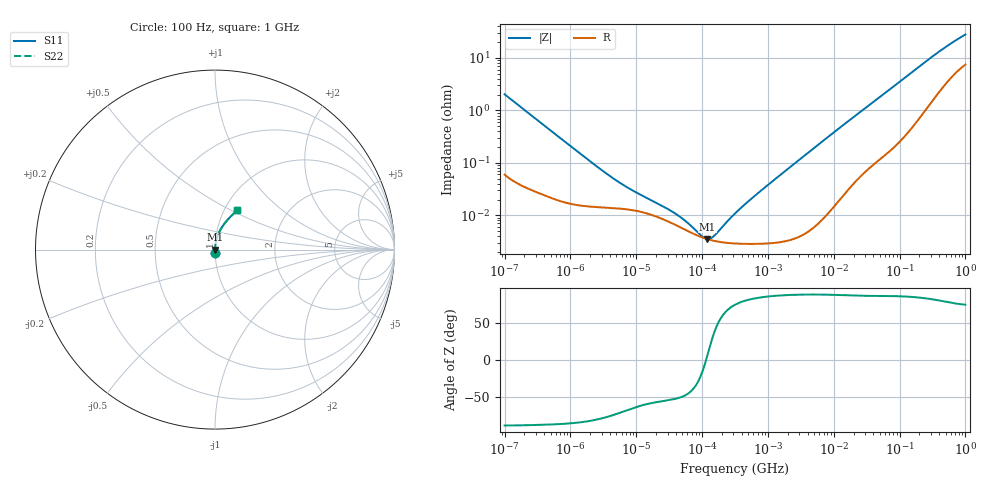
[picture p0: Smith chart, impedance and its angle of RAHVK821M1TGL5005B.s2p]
! RAHVK821M1TGL5005B  S-PARAMETER MODEL  (AEC-Q200 qualified)
! Model Generated by ELNA Corporation (http://www.ty-top.com)
! Version 1.0
! ELNA Control No. 201211
! Copyright (c) 2020 ELNA CO.,LTD. All Rights Reserved.
! Products Name : CONDUCTIVE POLYMER HYBRID ALUMINUM ELECTROLYTIC CAPACITORS
! Characteristics :
!  Capacitance  :  820uF  ,  Rated voltage  :  25V
!  Operating Temp. Range  :  -55 to +125 degC  ,  Endurance  :  6000hr at 125 degC
!  Dimension D  :  12.5mm  ,  Dimension L  :  13.5mm
! Frequency Range : 100Hz - 1GHz
! External Node Assignments :
!  1  o---| |---o  2
# MHz S RI R 50
!Freq[MHz].  S11 Real  S11 Imag  S21 Real  S21 Imag  S12 Real  S12 Imag  S22 Real  S22 Imag
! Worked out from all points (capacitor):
!   401 points, 100 Hz to 1 GHz, reference 50 ohm
!   read as one part in series: C = 782 uF near 108 Hz
!   lowest |Z| = 3.53 mohm at 120.2 kHz (marker M1)
!   series resonance near 115 kHz, so ESL is about 2.4 nH
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0.0001  0.00101 -0.0203  0.999 0.0203  0.999 0.0203  0.00101 -0.0203
0.000113  0.000853 -0.018  0.9991 0.018  0.9991 0.018  0.000853 -0.018
0.001488  0.000154 -0.00141  0.9998 0.00141  0.9998 0.00141  0.000154 -0.00141
0.00333  0.000141 -0.000642  0.9999 0.000642  0.9999 0.000642  0.000141 -0.000642
0.005855  0.000134 -0.000381  0.9999 0.000381  0.9999 0.000381  0.000134 -0.000381
0.009495  0.000123 -0.000254  0.9999 0.000254  0.9999 0.000254  0.000123 -0.000254
0.022131  9.04e-05 -0.000136  0.9999 0.000136  0.9999 0.000136  9.04e-05 -0.000136
0.040504  6.44e-05 -8.28e-05  0.9999 8.28e-05  0.9999 8.28e-05  6.44e-05 -8.28e-05
0.043904  6.13e-05 -7.64e-05  0.9999 7.64e-05  0.9999 7.64e-05  6.13e-05 -7.64e-05
0.120226  3.51e-05 3.68e-06  1 -3.68e-06  1 -3.68e-06  3.51e-05 3.68e-06
0.269153  2.94e-05 8.33e-05  1 -8.33e-05  1 -8.33e-05  2.94e-05 8.33e-05
0.291743  2.92e-05 9.35e-05  1 -9.35e-05  1 -9.35e-05  2.92e-05 9.35e-05
0.316228  2.9e-05 0.000104  1 -0.000104  1 -0.000104  2.9e-05 0.000104
0.473151  2.85e-05 0.00017  1 -0.00017  1 -0.00017  2.85e-05 0.00017
0.767361  2.87e-05 0.000287  1 -0.000287  1 -0.000287  2.87e-05 0.000287
4.704354  5.86e-05 0.0018  0.9999 -0.0018  0.9999 -0.0018  5.86e-05 0.0018
15.13561  0.0003 0.00569  0.9997 -0.00569  0.9997 -0.00569  0.0003 0.00569
69.9842  0.00225 0.0247  0.9977 -0.0247  0.9977 -0.0247  0.00225 0.0247
169.8244  0.00879 0.058  0.9912 -0.058  0.9912 -0.058  0.00879 0.058
365.1741  0.0326 0.1145  0.9674 -0.1145  0.9674 -0.1145  0.0326 0.1145
641.9482  0.0752 0.1716  0.9248 -0.1716  0.9248 -0.1716  0.0752 0.1716
1000  0.125 0.2204  0.875 -0.2204  0.875 -0.2204  0.125 0.2204
